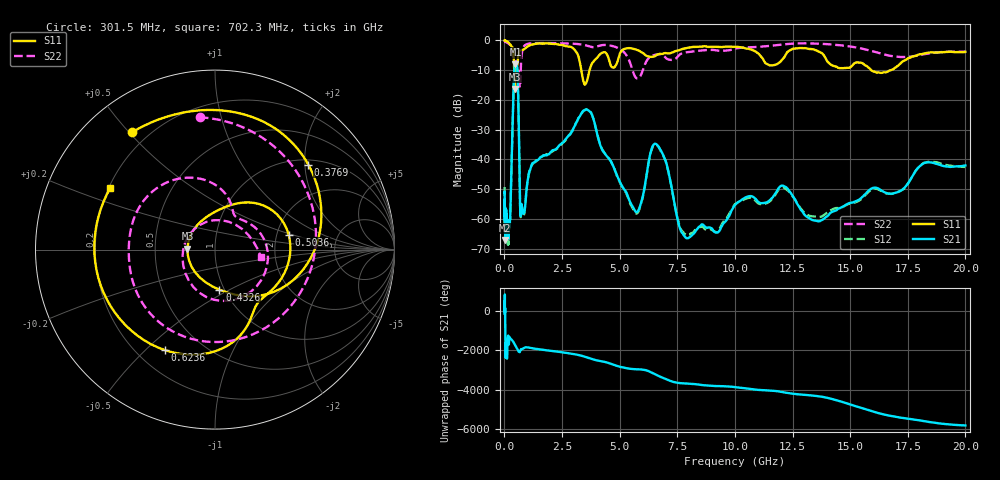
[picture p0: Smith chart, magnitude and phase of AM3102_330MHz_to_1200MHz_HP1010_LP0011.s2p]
! Date/Time: Tue, Sep 11, 2018 5:19 PM
! Network Analyzer: Agilent Technologies E8362B Rev: A.07.50.63
! Sweep from 0.010 to 20.000 GHz, 1601 Points, Sweep Type: LOG
! Power Supply: 4.949 V, 0.001 A
# Hz S DB R 50
!freq MagS11 AngS11 MagS21 AngS21 MagS12 AngS12 MagS22 AngS22
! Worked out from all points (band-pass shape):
!   1601 points, 10 MHz to 20 GHz, reference 50 ohm
!   highest |S21| = -7.97 dB at 478 MHz (marker M1); lowest = -67.0 dB at 41.98 MHz (marker M2)
!   |S21| within 3 dB of the highest: 424.5 MHz to 569 MHz (144.5 MHz wide, 29.1 % of centre)
!   lowest |S11| = -16.3 dB at 449.3 MHz (marker M3), VSWR 1.36, Z = 36.7 + j0.421 ohm
!   |S11| at or under -10 dB: 425.4 MHz to 477 MHz (51.61 MHz wide, 11.4 % of centre); 3.338 GHz to 3.694 GHz (356.5 MHz wide, 10.1 % of centre); 15.91 GHz to 16.76 GHz (850.7 MHz wide, 5.21 % of centre)
!   |S22| runs from -15.8 to -0.2 dB; largest |S21 - S12| = 0.005
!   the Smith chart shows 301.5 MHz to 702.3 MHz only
!   S11 on the Smith chart (normalised r, x): 301.5 MHz: 0.14, +0.51; 376.9 MHz: 1.11, +2.08; 432.6 MHz: 0.95, -0.45; 503.6 MHz: 2.33, +0.46; 623.6 MHz: 0.31, -0.58; 702.3 MHz: 0.21, +0.26
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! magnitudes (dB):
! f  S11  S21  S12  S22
! 10 MHz  0.0  -51.2  -49.2  -0.2
! 35.55 MHz  0.0  -64.4  -61.2  -0.3
! 41.98 MHz  0.0  -67.0  -65.1  -0.4
! 126.4 MHz  -0.4  -63.8  -62.0  -0.8
! 168.9 MHz  -0.6  -65.2  -68.2  -1.0
! 301.5 MHz  -1.9  -45.0  -45.1  -2.6
! 376.9 MHz  -3.1  -21.8  -21.8  -5.6
! 432.6 MHz  -13.0  -9.9  -9.9  -6.1
! 447.2 MHz  -16.2  -8.6  -8.7  -6.3
! 449.3 MHz  -16.3  -8.5  -8.6  -6.4
! 478 MHz  -9.8  -8.0  -8.1  -6.3
! 503.6 MHz  -7.6  -8.0  -8.0  -7.0
! 569.8 MHz  -7.7  -11.1  -11.2  -13.2
! 623.6 MHz  -4.1  -28.0  -28.0  -10.4
! 702.3 MHz  -3.4  -59.0  -59.2  -11.7
! 1.59 GHz  -1.0  -39.2  -39.1  -0.9
! 3.617 GHz  -12.7  -23.4  -23.1  -1.8
! 5.652 GHz  -2.9  -57.1  -57.7  -11.9
! 6.58 GHz  -5.0  -34.8  -35.0  -4.8
! 7.958 GHz  -2.4  -66.5  -65.5  -3.9
! 13.68 GHz  -3.9  -60.8  -59.3  -1.1
! 20 GHz  -3.9  -42.0  -42.5  -3.7
